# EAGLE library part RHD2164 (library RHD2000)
Intan Technologies RHD2164 chip
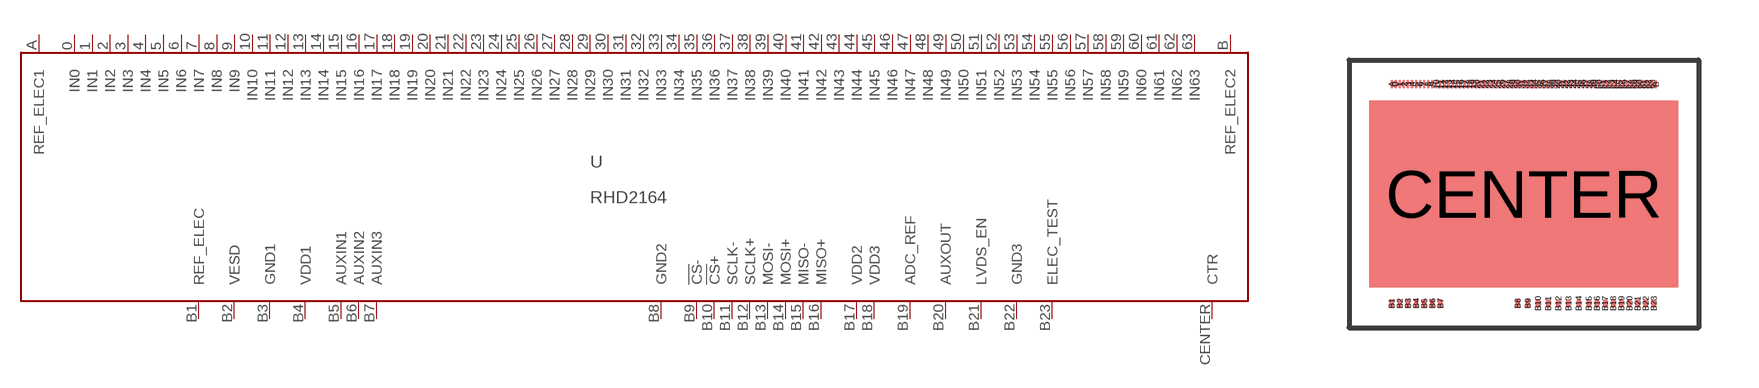
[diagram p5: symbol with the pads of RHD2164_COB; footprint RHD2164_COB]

Designator prefix U

## RHD2164_COB  [RHD2164_COB]
0  IN0  in
1  IN1  in
2  IN2  in
3  IN3  in
4  IN4  in
5  IN5  in
6  IN6  in
7  IN7  in
8  IN8  in
9  IN9  in
10  IN10  in
11  IN11  in
12  IN12  in
13  IN13  in
14  IN14  in
15  IN15  in
16  IN16  in
17  IN17  in
18  IN18  in
19  IN19  in
20  IN20  in
21  IN21  in
22  IN22  in
23  IN23  in
24  IN24  in
25  IN25  in
26  IN26  in
27  IN27  in
28  IN28  in
29  IN29  in
30  IN30  in
31  IN31  in
32  IN32  in
33  IN33  in
34  IN34  in
35  IN35  in
36  IN36  in
37  IN37  in
38  IN38  in
39  IN39  in
40  IN40  in
41  IN41  in
42  IN42  in
43  IN43  in
44  IN44  in
45  IN45  in
46  IN46  in
47  IN47  in
48  IN48  in
49  IN49  in
50  IN50  in
51  IN51  in
52  IN52  in
53  IN53  in
54  IN54  in
55  IN55  in
56  IN56  in
57  IN57  in
58  IN58  in
59  IN59  in
60  IN60  in
61  IN61  in
62  IN62  in
63  IN63  in
A  REF_ELEC1  in
B  REF_ELEC2  in
B1  REF_ELEC  in
B2  VESD  pwr
B3  GND1  pwr
B4  VDD1  pwr
B5  AUXIN1  in
B6  AUXIN2  in
B7  AUXIN3  in
B8  GND2  pwr
B9  !CS!-  in
B10  !CS!+  in
B11  SCLK-  in
B12  SCLK+  in
B13  MOSI-  in
B14  MOSI+  in
B15  MISO-  out
B16  MISO+  out
B17  VDD2  pwr
B18  VDD3  pwr
B19  ADC_REF  pas
B20  AUXOUT  hiz
B21  LVDS_EN  in
B22  GND3  pwr
B23  ELEC_TEST  in
CENTER  CTR  pwr

## Footprint RHD2164_COB (pad centres in mm)
smd 0.051 x 0.203: 0 -3.2,2.743; 1 -3.099,2.743; 2 -2.997,2.743; 3 -2.896,2.743; 4 -2.794,2.743; 5 -2.692,2.743; 6 -2.591,2.743; 7 -2.489,2.743; 8 -2.388,2.743; 9 -2.286,2.743; 10 -2.184,2.743; 11 -2.083,2.743; 12 -1.981,2.743; 13 -1.88,2.743; 14 -1.778,2.743; 15 -1.676,2.743; 16 -1.575,2.743; 17 -1.473,2.743; 18 -1.372,2.743; 19 -1.27,2.743; 20 -1.168,2.743; 21 -1.067,2.743; 22 -0.965,2.743; 23 -0.864,2.743; 24 -0.762,2.743; 25 -0.66,2.743; 26 -0.559,2.743; 27 -0.457,2.743; 28 -0.356,2.743; 29 -0.254,2.743; 30 -0.152,2.743; 31 -0.051,2.743; 32 0.051,2.743; 33 0.152,2.743; 34 0.254,2.743; 35 0.356,2.743; 36 0.457,2.743; 37 0.559,2.743; 38 0.66,2.743; 39 0.762,2.743; 40 0.864,2.743; 41 0.965,2.743; 42 1.067,2.743; 43 1.168,2.743; 44 1.27,2.743; 45 1.372,2.743; 46 1.473,2.743; 47 1.575,2.743; 48 1.676,2.743; 49 1.778,2.743; 50 1.88,2.743; 51 1.981,2.743; 52 2.083,2.743; 53 2.184,2.743; 54 2.286,2.743; 55 2.388,2.743; 56 2.489,2.743; 57 2.591,2.743; 58 2.692,2.743; 59 2.794,2.743; 60 2.896,2.743; 61 2.997,2.743; 62 3.099,2.743; 63 3.2,2.743; A -3.302,2.743; B 3.302,2.743
smd 0.102 x 0.203: B1 -3.302,-2.743; B2 -3.099,-2.743; B3 -2.896,-2.743; B4 -2.692,-2.743; B5 -2.489,-2.743; B6 -2.286,-2.743; B7 -2.083,-2.743; B8 -0.152,-2.743; B9 0.102,-2.743; B10 0.356,-2.743; B11 0.61,-2.743; B12 0.864,-2.743; B13 1.118,-2.743; B14 1.372,-2.743; B15 1.626,-2.743; B16 1.829,-2.743; B17 2.032,-2.743; B18 2.235,-2.743; B19 2.438,-2.743; B20 2.642,-2.743; B21 2.845,-2.743; B22 3.048,-2.743; B23 3.251,-2.743
smd 7.722 x 4.674: CENTER 0,0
